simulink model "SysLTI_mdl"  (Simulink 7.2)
settings: Solver=ode45  StartTime=0.0  StopTime=10.0  RelTol=1e-3
libraries: cstblocks x1

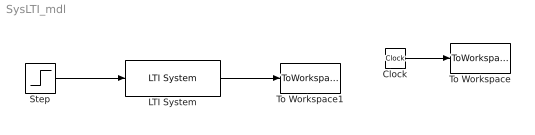
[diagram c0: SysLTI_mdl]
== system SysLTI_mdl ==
  Clock : Clock
  LTI System : cstblocks/LTI System  SystemSampleTime=-1  sys=sys  IC=X0
  Step : Step  SampleTime=0
  To Workspace : ToWorkspace  VariableName=time  SampleTime=-1  SaveFormat=Array
  To Workspace1 : ToWorkspace  VariableName=y  SampleTime=-1  SaveFormat=Array
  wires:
  Step/1 -> LTI System/1
  Clock/1 -> To Workspace/1
  LTI System/1 -> To Workspace1/1
